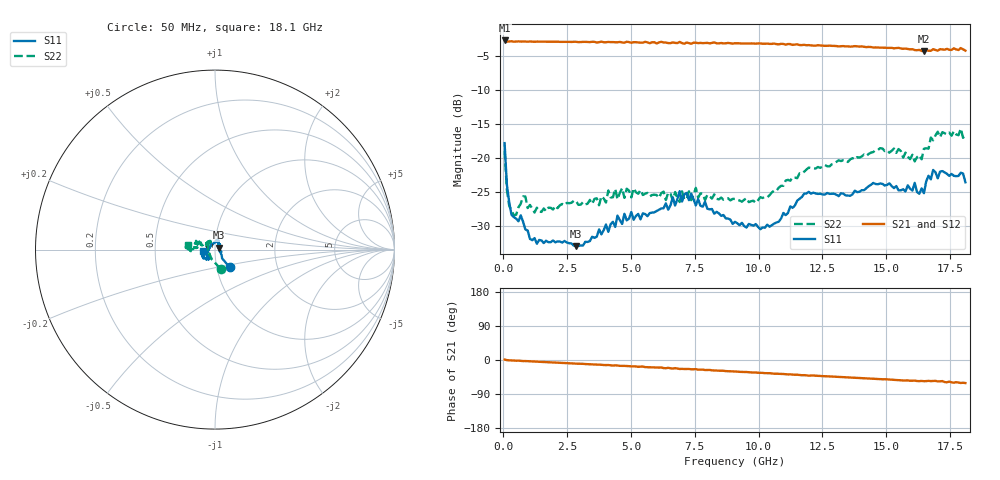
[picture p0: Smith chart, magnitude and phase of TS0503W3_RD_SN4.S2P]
! Network Analyzer HP8720D.06.14 Serial No. US36140669
! 30 Sep 2005  12:14:51
! Frequency  S11  S21  S12  S22
# HZ  S  DB R 50
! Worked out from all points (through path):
!   201 points, 50 MHz to 18.1 GHz, reference 50 ohm
!   highest |S21| = -2.66 dB at 50 MHz (marker M1); lowest = -4.3 dB at 16.48 GHz (marker M2)
!   group delay of S21, straight-line fit = 9.44 ps
!   lowest |S11| = -33.0 dB at 2.848 GHz (marker M3), VSWR 1.05, Z = 52 + j1.13 ohm
!   |S11| at or under -10 dB: start of sweep to end of sweep
!   |S22| runs from -28.4 to -15.7 dB; largest |S21 - S12| = 0.022
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5e7  -17.80 -50.3  -2.66 1.1  -2.70 1.1  -18.93 -73.2
1.4025e8  -23.99 -51.1  -2.83 -0.3  -2.77 -0.4  -24.75 -107.3
3.2075e8  -28.38 -32.9  -2.78 -1.0  -2.79 -1.1  -27.71 -134.2
7.72e8  -29.37 -19.4  -2.81 -2.8  -2.81 -2.7  -25.66 -167.7
1.3135e9  -32.64 -1.9  -2.82 -4.5  -2.81 -4.3  -27.32 171.8
2.84775e9  -32.99 28.9  -2.86 -9.6  -2.86 -9.5  -26.30 147.5
3.1185e9  -32.91 15.7  -2.87 -10.1  -2.86 -10.4  -26.51 160.3
4.382e9  -30.17 38.9  -2.93 -14.1  -2.86 -14.5  -24.55 146.3
4.47225e9  -28.48 37.5  -2.93 -14.5  -2.90 -14.2  -26.08 149.3
4.65275e9  -29.72 39.6  -2.96 -15.3  -2.86 -15.2  -24.45 147.8
6.09675e9  -27.64 60.4  -2.95 -20.0  -2.85 -19.7  -25.86 135.3
6.7285e9  -27.00 74.1  -3.02 -21.5  -3.10 -22.0  -25.01 123.0
6.909e9  -24.88 76.0  -2.87 -23.6  -2.93 -22.9  -26.49 120.1
7.54075e9  -26.99 73.1  -3.00 -24.2  -2.87 -25.0  -24.40 128.6
9.075e9  -29.41 110.1  -3.07 -30.4  -3.02 -30.2  -26.03 127.9
1.042875e10  -30.13 160.2  -3.16 -34.8  -3.10 -35.1  -25.48 141.7
1.21435e10  -25.11 -155.2  -3.42 -40.8  -3.36 -40.7  -21.52 159.2
1.512175e10  -23.73 -124.1  -3.75 -51.7  -3.66 -51.0  -19.21 161.0
1.61145e10  -23.65 -130.2  -4.08 -54.4  -3.91 -55.0  -20.49 165.8
1.64755e10  -25.18 -124.7  -4.26 -56.0  -4.18 -54.5  -18.63 173.1
1.68365e10  -21.76 -143.8  -3.95 -55.4  -4.07 -55.9  -17.38 -176.2
1.81e10  -23.58 -171.6  -4.16 -60.8  -4.09 -62.0  -16.45 171.0
